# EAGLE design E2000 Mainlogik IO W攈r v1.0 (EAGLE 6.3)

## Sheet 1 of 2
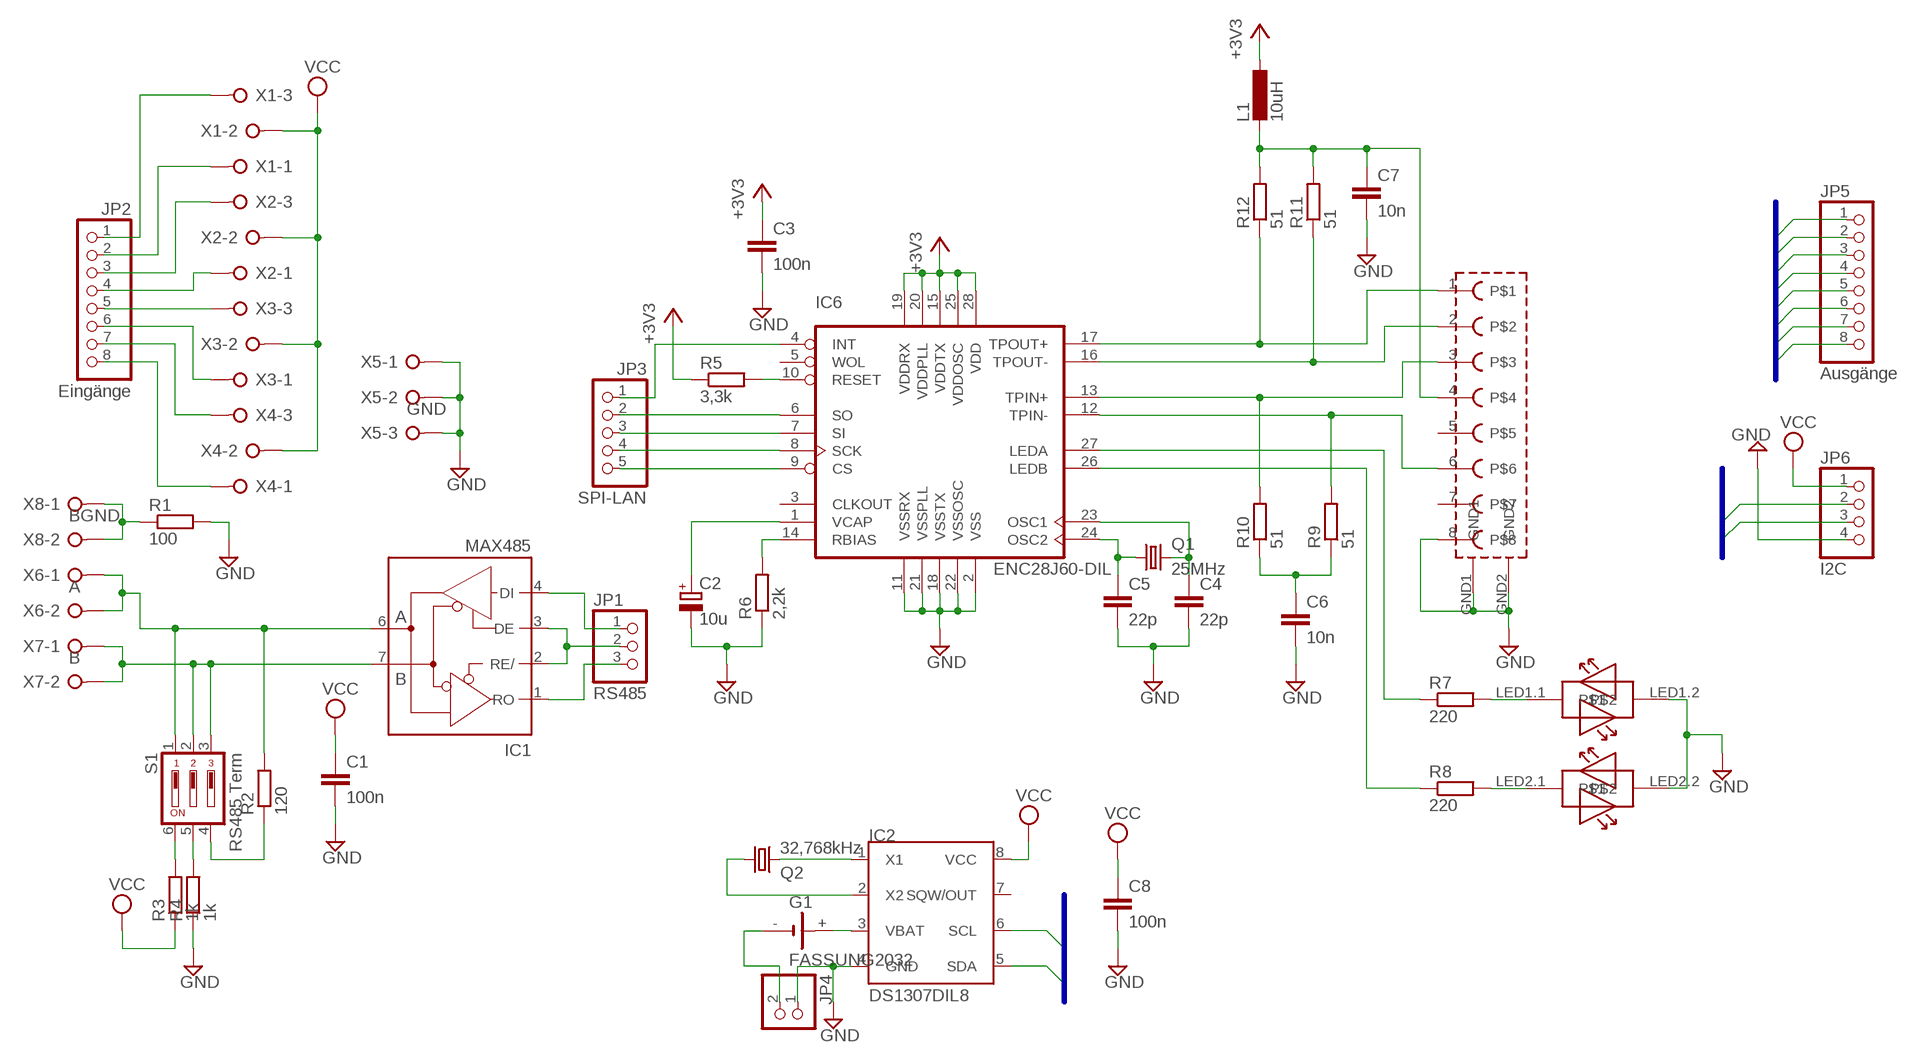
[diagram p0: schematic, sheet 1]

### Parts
C1  100n  C-EU050-025X075  [C050-025X075]
C2  10u  CPOL-EUE5-6  [E5-6]
C3  100n  C-EUC1206  [C1206]
C4  22p  C-EUC1206  [C1206]
C5  22p  C-EUC1206  [C1206]
C6  10n  C-EUC1206  [C1206]
C7  10n  C-EUC1206  [C1206]
C8  100n  C-EU050-025X075  [C050-025X075]
G1  FASSUNG2032  [BATTERY_1236_C]
IC1  MAX485  MAX481CPA  [DIL08]
IC2  DS1307DIL8  [DIL08]
IC6  ENC28J60-DIL  [DIL28-3]
J4  MAGJACK  [MAGJACK]
JP1  RS485  PINHD-1X3  [1X03]
JP2  Eingänge  PINHD-1X8  [1X08]
JP3  SPI-LAN  PINHD-1X5  [1X05]
JP4  PINHD-1X2  [1X02]
JP5  Ausgänge  PINHD-1X8  [1X08]
JP6  I2C  PINHD-1X4  [1X04]
L1  10uH  L-EUL1206  [C1206]
Q1  25MHz  CRYSTALHC49S  [HC49/S]
Q2  32,768kHz  CRYSTALTC38H  [TC38H]
R1  100  R-EU_0207/10  [0207/10]
R2  120  R-EU_0207/10  [0207/10]
R3  1k  R-EU_0207/10  [0207/10]
R4  1k  R-EU_0207/10  [0207/10]
R5  3,3k  R-EU_R1206  [R1206]
R6  2,2k  R-EU_R1206  [R1206]
R7  220  R-EU_R1206  [R1206]
R8  220  R-EU_R1206  [R1206]
R9  51  R-EU_R1206  [R1206]
R10  51  R-EU_R1206  [R1206]
R11  51  R-EU_R1206  [R1206]
R12  51  R-EU_R1206  [R1206]
S1  RS485 Term  DIP03YL  [DIP03YL]
X1  W237-3E  [W237-3E]
X2  W237-3E  [W237-3E]
X3  W237-3E  [W237-3E]
X4  W237-3E  [W237-3E]
X5  GND  W237-3E  [W237-3E]
X6  A  W237-02P  [W237-132]
X7  B  W237-02P  [W237-132]
X8  BGND  W237-02P  [W237-132]

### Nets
+3V3: C3.1 IC6.15(VDDTX) IC6.19(VDDRX) IC6.20(VDDPLL) IC6.25(VDDOSC) IC6.28(VDD) L1.1 R5.1 ; also sheet 2
A1: JP5.1 ; also sheet 2
A2: JP5.2 ; also sheet 2
A3: JP5.3 ; also sheet 2
A4: JP5.4 ; also sheet 2
A5: JP5.5 ; also sheet 2
A6: JP5.6 ; also sheet 2
A7: JP5.7 ; also sheet 2
A8: JP5.8 ; also sheet 2
CS: IC6.9(CS) JP3.5
GND: C1.2 C2.- C3.2 C4.2 C5.2 C6.2 C7.2 C8.2 IC2.4(GND) IC6.2(VSS) IC6.11(VSSRX) IC6.18(VSSTX) IC6.21(VSSPLL) IC6.22(VSSOSC) J4.8 J4.GND1 J4.GND2 J4.LED1.2 J4.LED2.2 JP4.1 JP6.4 R1.2 R4.1 R6.1 X5.1 X5.2 X5.3 ; also sheet 2
INT: IC6.4(INT) JP3.1
MISO: IC6.6(SO) JP3.2
MOSI: IC6.7(SI) JP3.3
N$1: R1.1 X8.1 X8.2
N$2: IC1.6(A) R2.2 S1.1 X6.1 X6.2
N$3: IC1.7(B) S1.2 S1.3 X7.1 X7.2
N$4: R2.1 S1.4
N$5: IC2.1(X1) Q2.2
N$6: R4.2 S1.5
N$7: R3.2 S1.6
N$8: IC2.2(X2) Q2.1
N$9: G1.+ IC2.3(VBAT)
N$10: JP2.5 X3.3
N$11: JP2.4 X2.1
N$12: JP2.3 X2.3
N$13: JP2.2 X1.1
N$14: JP2.1 X1.3
N$15: JP2.6 X3.1
N$16: JP2.7 X4.3
N$17: JP2.8 X4.1
N$18: G1.- JP4.2
N$19: IC6.10(RESET) R5.2
N$25: IC6.14(RBIAS) R6.2
N$26: C2.+ IC6.1(VCAP)
N$28: C5.1 IC6.24(OSC2) Q1.1
N$29: C4.1 IC6.23(OSC1) Q1.2
N$32: C7.1 J4.4 L1.2 R11.2 R12.2
N$33: IC6.13(TPIN+) J4.3 R10.2
N$34: J4.LED1.1 R7.2
N$35: J4.LED2.1 R8.2
N$36: IC6.12(TPIN-) J4.6 R9.2
N$37: IC6.27(LEDA) R7.1
N$38: IC6.26(LEDB) R8.1
N$41: IC6.16(TPOUT-) J4.2 R11.1
N$42: IC6.17(TPOUT+) J4.1 R12.1
N$43: C6.1 R9.1 R10.1
RX: IC1.1(RO) JP1.3
SCK: IC6.8(SCK) JP3.4
SCL: IC2.6(SCL) JP6.2 ; also sheet 2
SDA: IC2.5(SDA) JP6.3 ; also sheet 2
SEL: IC1.2(RE/) IC1.3(DE) JP1.2
TX: IC1.4(DI) JP1.1
VCC: C1.1 C8.1 IC2.8(VCC) JP6.1 R3.1 X1.2 X2.2 X3.2 X4.2 ; also sheet 2
Unconnected: IC2.7(SQW/OUT) IC6.3(CLKOUT) IC6.5(WOL) J4.5 J4.7

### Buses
SCL,SDA
A1,A2,A3,A4,A5,A6,A7,A8

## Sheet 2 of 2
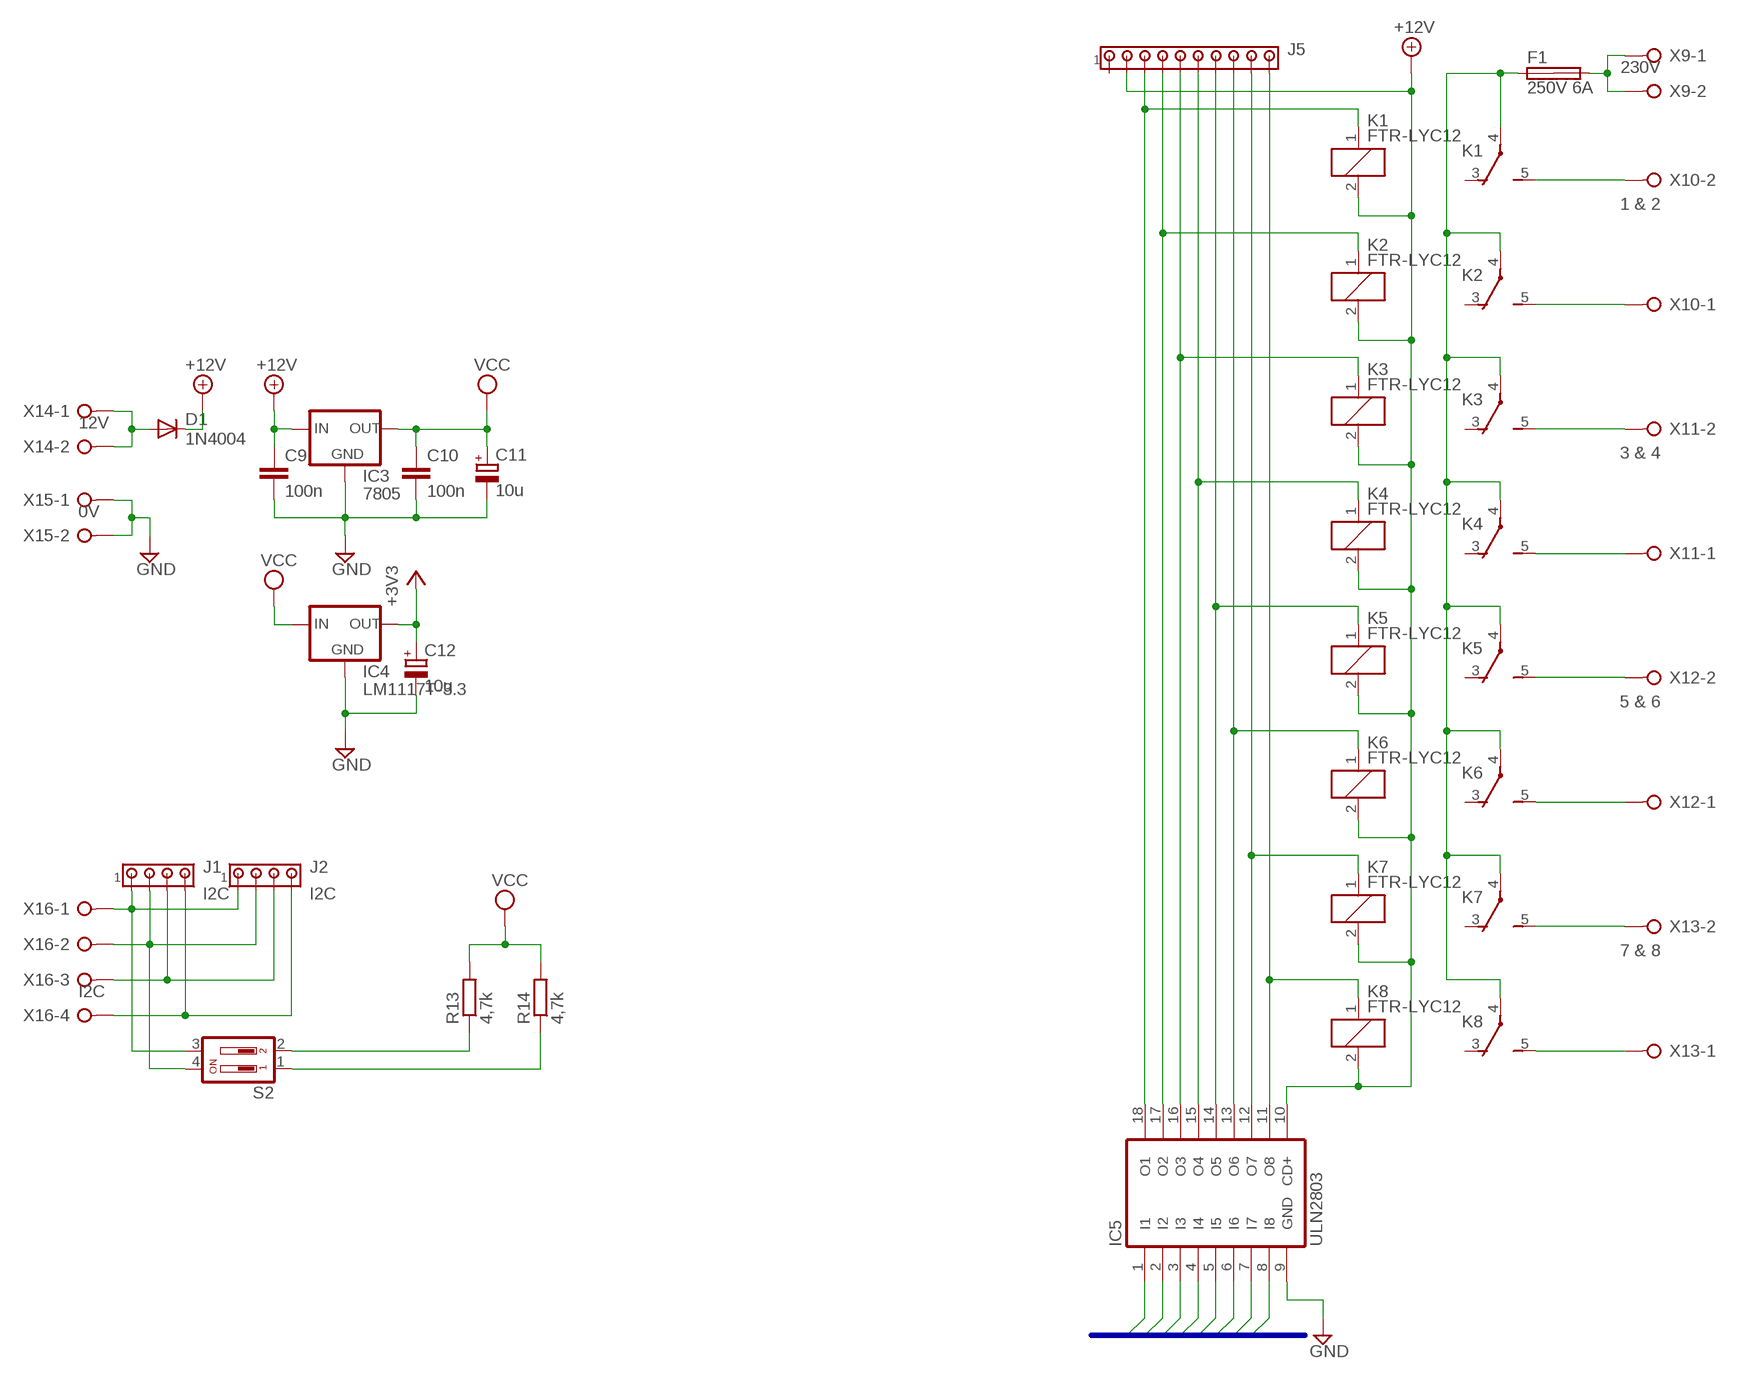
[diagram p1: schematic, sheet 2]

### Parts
C9  100n  C-EU050-025X075  [C050-025X075]
C10  100n  C-EU050-025X075  [C050-025X075]
C11  10u  CPOL-EUE5-6  [E5-6]
C12  10u  CPOL-EUE5-6  [E5-6]
D1  1N4004  [DO41-10]
F1  250V 6A  SHK20L  [SHK20L]
IC3  7805  78XXL  [78XXL]
IC4  LM1117T-3.3  [TO220]
IC5  ULN2803  ULN2803A  [DIL18]
J1  I2C  MTA04-100  [10X04MTA]
J2  I2C  MTA04-100  [10X04MTA]
J5  MTA10-100  [10X10MTA]
K1  FTR-LYC12  [FTR-LYC]
K2  FTR-LYC12  [FTR-LYC]
K3  FTR-LYC12  [FTR-LYC]
K4  FTR-LYC12  [FTR-LYC]
K5  FTR-LYC12  [FTR-LYC]
K6  FTR-LYC12  [FTR-LYC]
K7  FTR-LYC12  [FTR-LYC]
K8  FTR-LYC12  [FTR-LYC]
R13  4,7k  R-EU_0207/10  [0207/10]
R14  4,7k  R-EU_0207/10  [0207/10]
S2  DIP02YL  [DIP02YL]
X9  230V  W237-02P  [W237-132]
X10  1 & 2  W237-02P  [W237-132]
X11  3 & 4  W237-02P  [W237-132]
X12  5 & 6  W237-02P  [W237-132]
X13  7 & 8  W237-02P  [W237-132]
X14  12V  W237-02P  [W237-132]
X15  0V  W237-02P  [W237-132]
X16  I2C  W237-04P  [W237-4P]

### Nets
+3V3: C12.+ IC4.2(OUT) ; also sheet 1
+12V: C9.1 D1.C IC3.IN IC5.10(CD+) J5.2 K1.2 K2.2 K3.2 K4.2 K5.2 K6.2 K7.2 K8.2
A1: IC5.1(I1) ; also sheet 1
A2: IC5.2(I2) ; also sheet 1
A3: IC5.3(I3) ; also sheet 1
A4: IC5.4(I4) ; also sheet 1
A5: IC5.5(I5) ; also sheet 1
A6: IC5.6(I6) ; also sheet 1
A7: IC5.7(I7) ; also sheet 1
A8: IC5.8(I8) ; also sheet 1
GND: C9.2 C10.2 C11.- C12.- IC3.GND IC4.1(GND) IC5.9(GND) J1.4 J2.4 X15.1 X15.2 X16.4 ; also sheet 1
N$20: F1.2A X9.1 X9.2
N$21: F1.1A K1.4(-1:P) K2.4(-1:P) K3.4(-1:P) K4.4(-1:P) K5.4(-1:P) K6.4(-1:P) K7.4(-1:P) K8.4(-1:P)
N$22: K1.5(-1:S) X10.2
N$23: K2.5(-1:S) X10.1
N$24: K8.5(-1:S) X13.1
N$27: K7.5(-1:S) X13.2
N$30: K6.5(-1:S) X12.1
N$31: K5.5(-1:S) X12.2
N$39: K4.5(-1:S) X11.1
N$40: K3.5(-1:S) X11.2
N$44: D1.A X14.1 X14.2
N$45: IC5.11(O8) J5.10 K8.1
N$46: IC5.12(O7) J5.9 K7.1
N$47: IC5.13(O6) J5.8 K6.1
N$48: IC5.14(O5) J5.7 K5.1
N$49: IC5.15(O4) J5.6 K4.1
N$50: IC5.16(O3) J5.5 K3.1
N$51: IC5.17(O2) J5.4 K2.1
N$52: IC5.18(O1) J5.3 K1.1
N$53: R13.1 S2.2
N$54: R14.1 S2.1
SCL: J1.1 J2.1 S2.3 X16.1 ; also sheet 1
SDA: J1.2 J2.2 S2.4 X16.2 ; also sheet 1
VCC: C10.1 C11.+ IC3.OUT IC4.3(IN) J1.3 J2.3 R13.2 R14.2 X16.3 ; also sheet 1
Unconnected: F1.1B F1.2B J5.1 K1.3(-1:O) K2.3(-1:O) K3.3(-1:O) K4.3(-1:O) K5.3(-1:O) K6.3(-1:O) K7.3(-1:O) K8.3(-1:O)

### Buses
A1,A2,A3,A4,A5,A6,A7,A8

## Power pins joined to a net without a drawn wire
GND: IC1.5(GND)
VCC: IC1.8(VCC)

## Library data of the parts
C1 C3-C10 = rcl:C-EU: CAPACITOR, European symbol
C2 C11 C12 = rcl:CPOL-EU: POLARIZED CAPACITOR, European symbol
D1 = diode:1N4004: DIODE
F1 = fuse:SHK20L: FUSE HOLDER 5 x 20 mm, SH contact, SHH1 Schukat, E1073 Buerklin; OC_FARNELL: unknown; OC_NEWARK: unknown
G1 = battery:FASSUNG2032: LI BATTERY Sonnenschein
IC1 = maxim:MAX481CPA: RS485 TRANSEIVER; MPN: MAX481CPA+; OC_FARNELL: unknown; OC_NEWARK: 99K3445
IC2 = dallas:DS1307: I2C Serial RTC w/56 bytes battery backed RAM
IC3 = v-reg:78XXL: VOLTAGE REGULATOR
IC4 = lm1117:LM1117T-*
IC5 = uln-udn:ULN2803A: DRIVER ARRAY
IC6 = enc28j60centered:ENC28J60-*: Microchip 10Mbit Ethernet controller with SPI interface Improved SOIC28 layout (pads in 0.01 raster, pin1 slightly smaller). Pin 6 (SO) changed from Out (paralleling several Outs gives an error) to OC. Author: Profi from mikrocontroller.net - forum Date: 2006.0827
J1 J2 = con-amp:MTA04-100: AMP connector
J4 = magjacksmalldrill:MAGJACK
J5 = con-amp:MTA10-100: AMP connector
JP1 = pinhead:PINHD-1X3: PIN HEADER
JP2 JP5 = pinhead:PINHD-1X8: PIN HEADER
JP3 = pinhead:PINHD-1X5: PIN HEADER
JP4 = pinhead:PINHD-1X2: PIN HEADER
JP6 = pinhead:PINHD-1X4: PIN HEADER
K1-K8 = relay:FTR-LYC: Schmales Netzrelais NETZRELAIS FTR-LYCA024V 1XUM 6A/250VAC Distributor: Conrad electronic Bestell Nr.: 504382 - 62 Source: http://www2.produktinfo.conrad.com/datenblaetter/500000-524999/504382-da-01-de-NETZRELAIS_FTR-LYCA024V_1XUM_6A_250VAC.pdf; OC_FARNELL: unknown; OC_NEWARK: unknown
L1 = rcl:L-EU: INDUCTOR, European symbol
Q1 = crystal:CRYSTAL: CRYSTAL; OC_FARNELL: 1667008; OC_NEWARK: unknown
Q2 = crystal:CRYSTAL: CRYSTAL; OC_FARNELL: unknown; OC_NEWARK: unknown
R1-R14 = rcl:R-EU_: RESISTOR, European symbol
S1 = switch-dil:DIP03YL: DIL/CODE SWITCH; OC_FARNELL: unknown; OC_NEWARK: unknown
S2 = switch-dil:DIP02YL: DIL/CODE SWITCH; OC_FARNELL: unknown; OC_NEWARK: unknown
X1-X5 = con-wago-508:W237-3E: WAGO SREW CLAMP; OC_FARNELL: unknown; OC_NEWARK: unknown
X6-X15 = con-wago-508:W237-02P: WAGO SREW CLAMP; OC_FARNELL: unknown; OC_NEWARK: unknown
X16 = con-wago-508:W237-04P: WAGO SREW CLAMP; OC_FARNELL: unknown; OC_NEWARK: unknown

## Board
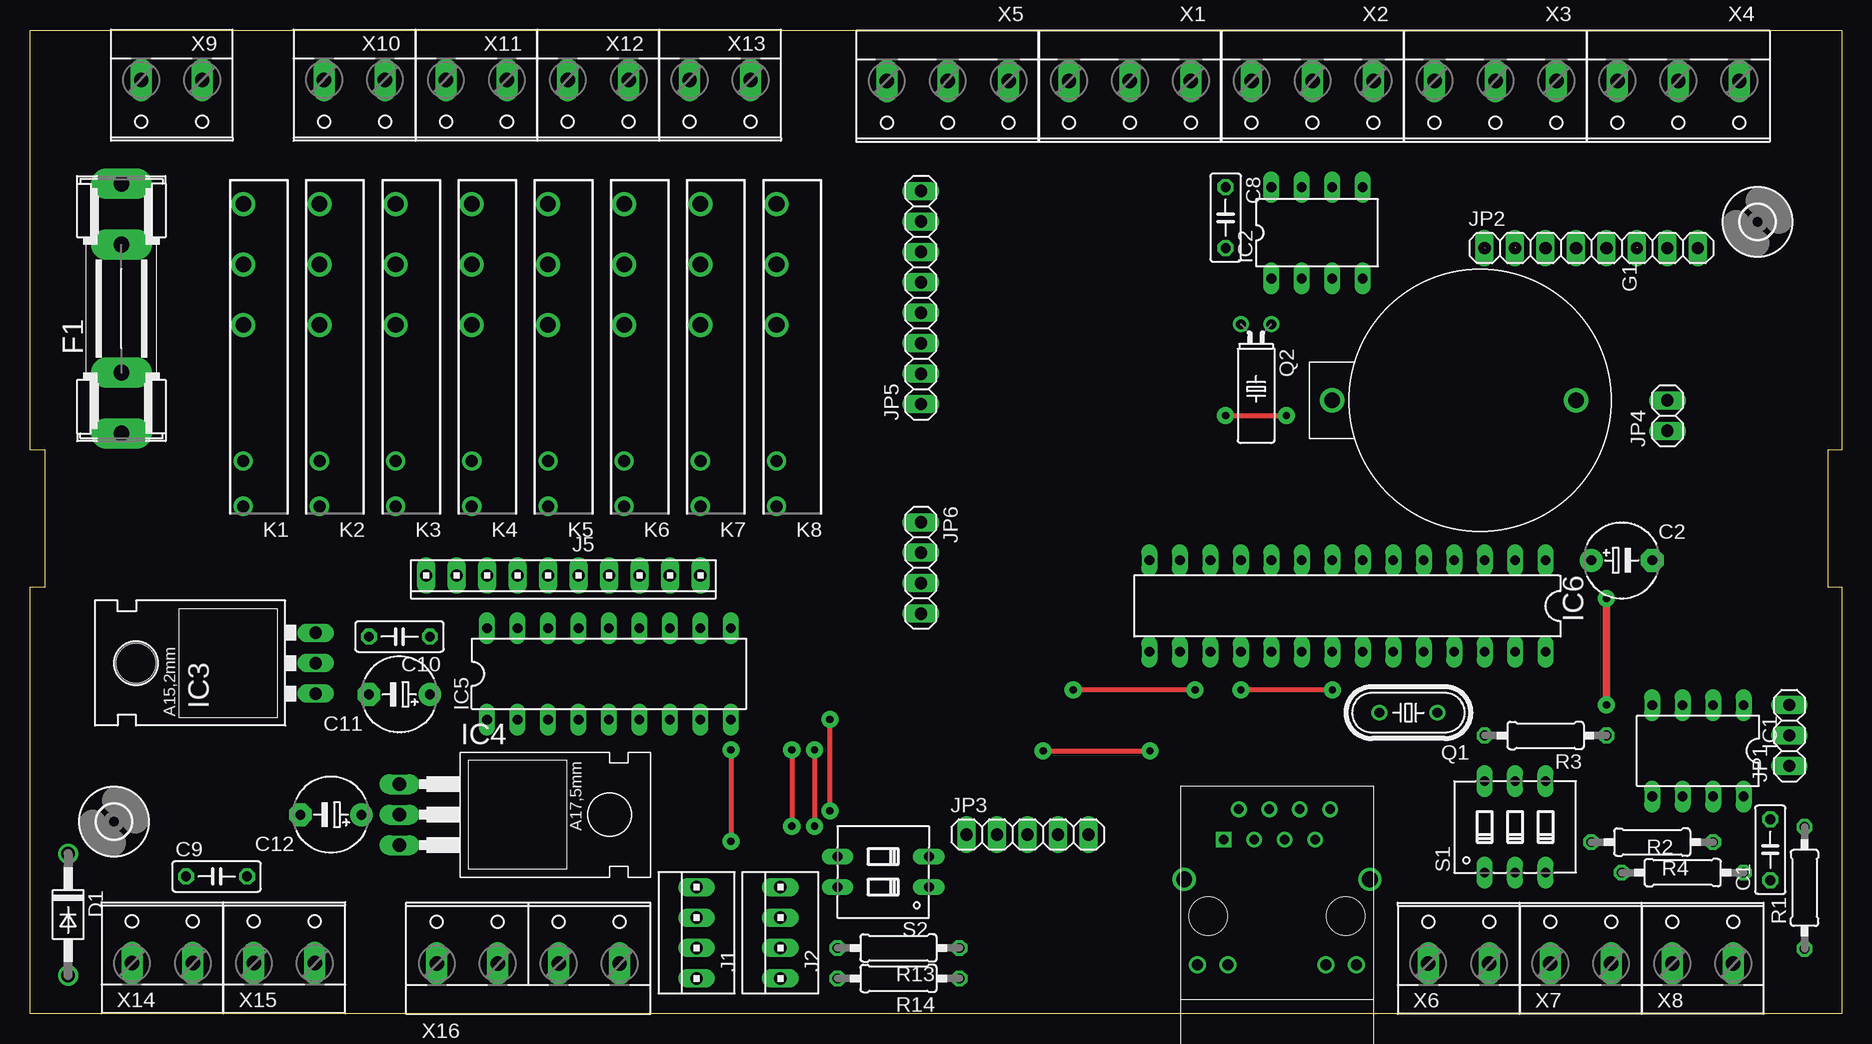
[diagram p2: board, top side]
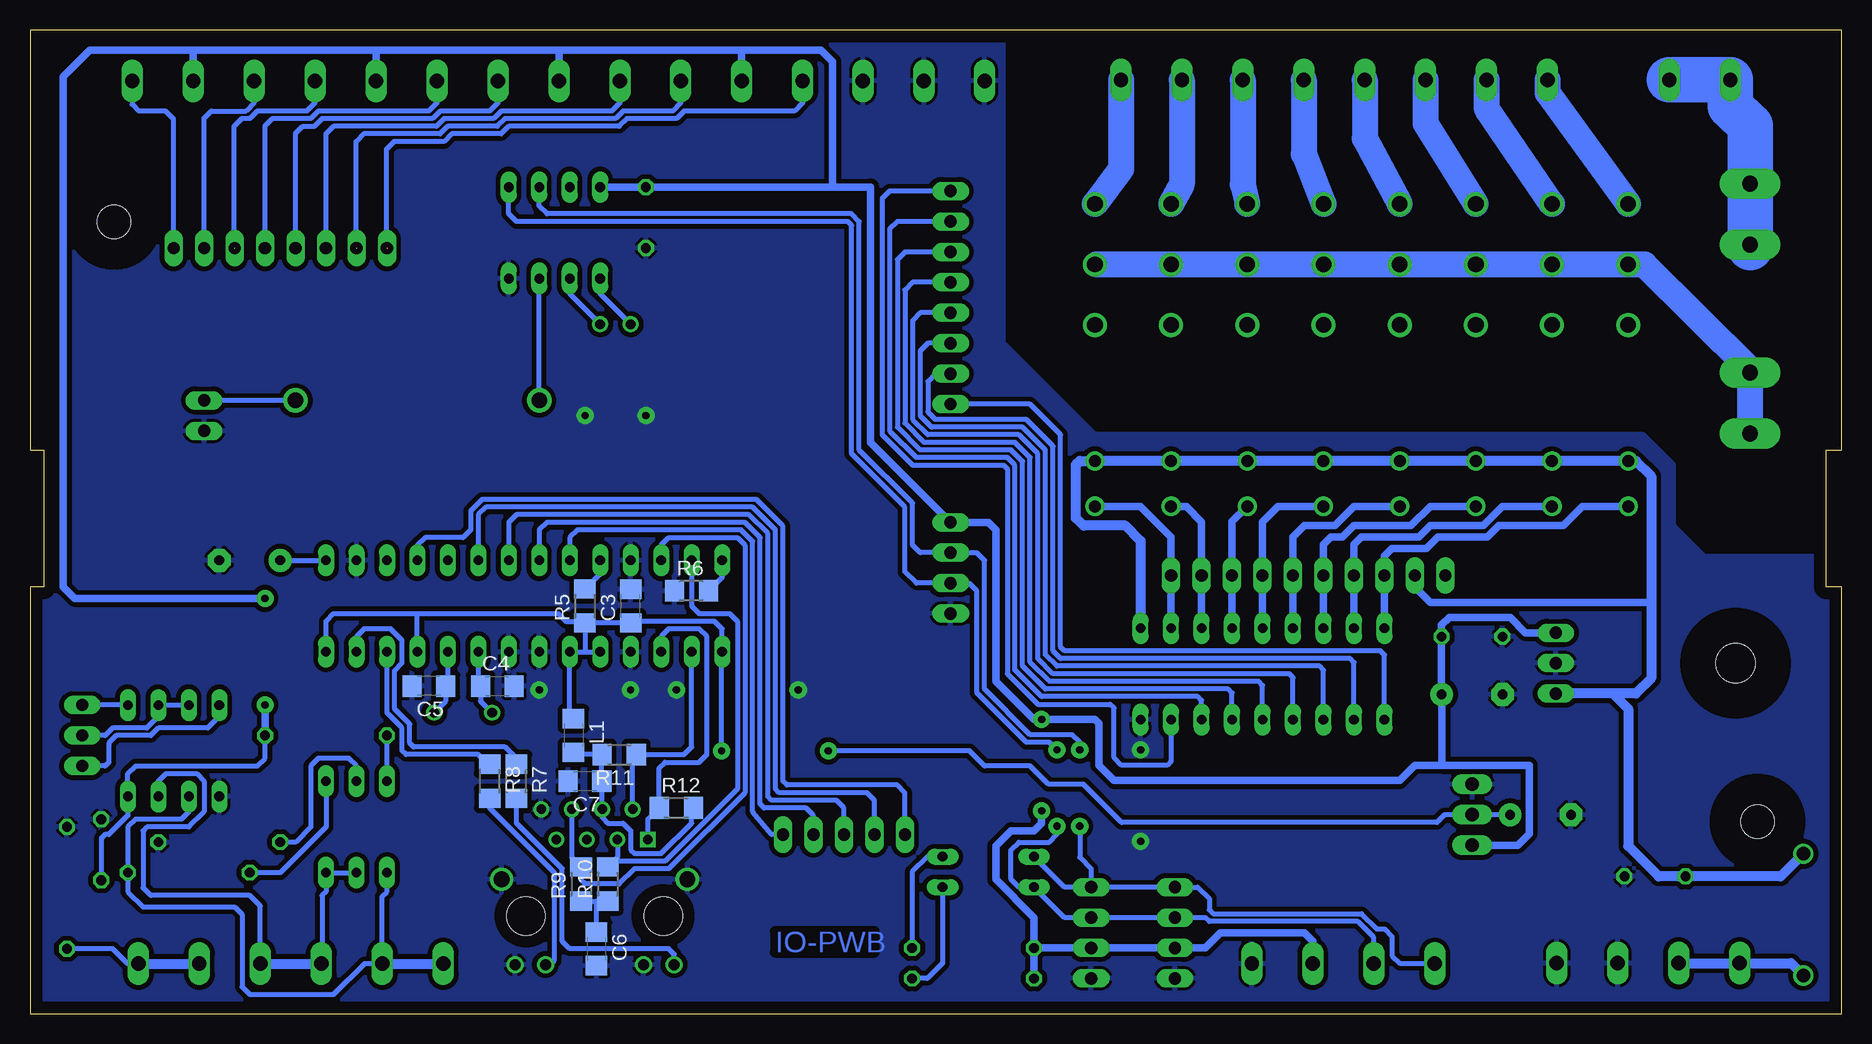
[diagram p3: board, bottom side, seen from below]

Size 151 x 82 mm. Coordinates in mm from the lower left corner, seen from the top.
Outline: 0,0 0,35.56 1.27,35.56 1.27,46.99 0,46.99 0,82 151,82 151,46.99 149.86,46.99 149.86,35.56 151,35.56 151,0 0,0
Copper layers (1*16): Top 0.035mm / dielectric 1.5mm / Bottom 0.035mm
Design rules "default": minimum track width 10mil, minimum drill 24mil, track to track 8mil, track to pad 8mil, pad to pad 8mil, via to via 8mil, smd to smd 8mil, copper to edge 40mil, drill to drill 8mil, minimum pad ring 10mil, minimum via ring 8mil, stop-mask expansion 4mil, vias tented up to drill 0mil, thermal gap 10mil

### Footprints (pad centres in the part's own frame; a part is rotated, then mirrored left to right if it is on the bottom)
C050-025X075 = drill 0.813 octagon: 1 -2.54,0; 2 2.54,0
E5-6 = drill 0.813 pad 1.905: + -2.54,0 | drill 0.813 pad 1.905 octagon: - 2.54,0
C1206 = smd 1.6 x 1.8: 1 -1.4,0; 2 1.4,0
DO41-10 = drill 1.118: A 5.08,0; C -5.08,0
SHK20L = drill 1.321 pad 2.54 long: 1A -10.414,0; 1B -5.334,0; 2A 10.414,0; 2B 5.334,0
BATTERY_1236_C = drill 1.27 pad 2.032: + 0,0; - 0,20.32
DIL08 = drill 0.813 long: 1 -3.81,-3.81; 2 -1.27,-3.81; 3 1.27,-3.81; 4 3.81,-3.81; 5 3.81,3.81; 6 1.27,3.81; 7 -1.27,3.81; 8 -3.81,3.81
78XXL = drill 1.016 long: GND 0,-3.81; IN -2.54,-3.81; OUT 2.54,-3.81 | hole 3.302: 0,11.176
TO220 = drill 1.118 long: 1 -2.54,-6.35; 2 0,-6.35; 3 2.54,-6.35
DIL18 = drill 0.813 long: 1 -10.16,-3.81; 2 -7.62,-3.81; 3 -5.08,-3.81; 4 -2.54,-3.81; 5 0,-3.81; 6 2.54,-3.81; 7 5.08,-3.81; 8 7.62,-3.81; 9 10.16,-3.81; 10 10.16,3.81; 11 7.62,3.81; 12 5.08,3.81; 13 2.54,3.81; 14 0,3.81; 15 -2.54,3.81; 16 -5.08,3.81; 17 -7.62,3.81; 18 -10.16,3.81
DIL28-3 = drill 0.813 long: 1 -16.51,-3.81; 2 -13.97,-3.81; 3 -11.43,-3.81; 4 -8.89,-3.81; 5 -6.35,-3.81; 6 -3.81,-3.81; 7 -1.27,-3.81; 8 1.27,-3.81; 9 3.81,-3.81; 10 6.35,-3.81; 11 8.89,-3.81; 12 11.43,-3.81; 13 13.97,-3.81; 14 16.51,-3.81; 15 16.51,3.81; 16 13.97,3.81; 17 11.43,3.81; 18 8.89,3.81; 19 6.35,3.81; 20 3.81,3.81; 21 1.27,3.81; 22 -1.27,3.81; 23 -3.81,3.81; 24 -6.35,3.81; 25 -8.89,3.81; 26 -11.43,3.81; 27 -13.97,3.81; 28 -16.51,3.81
10X04MTA = drill 1.016 long: 1 3.81,0; 2 1.27,0; 3 -1.27,0; 4 -3.81,0
MAGJACK = drill 0.8 square: 1 -4.445,6.35 | drill 0.8: 2 -3.175,8.89; 3 -1.905,6.35; 4 -0.635,8.89; 5 0.635,6.35; 6 1.905,8.89; 7 3.175,6.35; 8 4.445,8.89 | drill 1.3: GND1 -7.747,3.048; GND2 7.747,3.048 | drill 0.9: LED1.1 -6.629,-4.064; LED1.2 -4.089,-4.064; LED2.1 4.089,-4.064; LED2.2 6.629,-4.064 | hole 3.2: -5.715,0; 5.715,0
10X10MTA = drill 1.016 long: 1 11.43,0; 2 8.89,0; 3 6.35,0; 4 3.81,0; 5 1.27,0; 6 -1.27,0; 7 -3.81,0; 8 -6.35,0; 9 -8.89,0; 10 -11.43,0
1X03 = drill 1.016 long: 1 -2.54,0; 2 0,0; 3 2.54,0
1X08 = drill 1.016 long: 1 -8.89,0; 2 -6.35,0; 3 -3.81,0; 4 -1.27,0; 5 1.27,0; 6 3.81,0; 7 6.35,0; 8 8.89,0
1X05 = drill 1.016 long: 1 -5.08,0; 2 -2.54,0; 3 0,0; 4 2.54,0; 5 5.08,0
1X02 = drill 1.016 long: 1 -1.27,0; 2 1.27,0
1X04 = drill 1.016 long: 1 -3.81,0; 2 -1.27,0; 3 1.27,0; 4 3.81,0
FTR-LYC = drill 1 pad 1.6: 1 -3.78,0; 2 0,0 | drill 1.3 pad 2: 3 11.34,0; 4 16.38,0; 5 21.42,0
HC49/S = drill 0.813: 1 -2.413,0; 2 2.413,0
TC38H = drill 0.813: 1 -1.27,0; 2 1.27,0
0207/10 = drill 0.813 octagon: 1 -5.08,0; 2 5.08,0
R1206 = smd 1.6 x 1.803: 1 -1.422,0; 2 1.422,0
DIP03YL = drill 0.813 long: 1 -2.54,-3.81; 2 0,-3.81; 3 2.54,-3.81; 4 2.54,3.81; 5 0,3.81; 6 -2.54,3.81
DIP02YL = drill 0.813 long: 1 -1.27,-3.81; 2 1.27,-3.81; 3 1.27,3.81; 4 -1.27,3.81
2,8 = hole 2.8: 0,0
W237-3E = drill 1.194 long: 1 -5.08,-0.635; 2 0,-0.635; 3 5.08,-0.635
W237-132 = drill 1.194 long: 1 -2.54,-0.635; 2 2.54,-0.635
W237-4P = drill 1.194 long: 1 -7.62,-0.635; 2 -2.54,-0.635; 3 2.54,-0.635; 4 7.62,-0.635

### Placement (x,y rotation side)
C1  145.06,13.65 90 top
C2  132.68,37.78 0 top
C3  100.93,33.97 90 bottom
C4  112.04,27.3 0 bottom
C5  117.76,27.3 180 bottom
C6  103.79,5.4 270 bottom
C7  104.74,19.37 180 bottom
C8  99.66,66.36 270 top
C9  15.55,11.43 0 top
C10  30.8,31.43 180 top
C11  30.79,26.6 180 top
C12  25.08,16.57 180 top
D1  3.17,8.25 270 top
F1  7.62,58.77 90 top
G1  108.55,51.12 270 top
IC1  139.03,21.91 180 top
IC2  107.28,65.09 0 top
IC3  20.01,29.21 90 top
IC4  37.14,16.58 270 top
IC5  48.26,28.32 0 top
IC6  109.82,33.97 180 top
J1  55.56,6.73 90 top
J2  62.55,6.73 90 top
J4  103.94,8.14 0 top
J5  44.45,36.51 180 top
JP1  146.65,23.18 90 top
JP2  130.14,63.82 0 top
JP3  83.15,14.92 0 top
JP4  136.49,49.85 90 top
JP5  74.26,59.69 90 top
JP6  74.26,37.15 270 top
K1  17.78,46.07 90 top
K2  24.13,46.07 90 top
K3  30.48,46.07 90 top
K4  36.83,46.07 90 top
K5  43.18,46.07 90 top
K6  49.53,46.07 90 top
K7  55.88,46.07 90 top
K8  62.23,46.07 90 top
L1  105.69,23.18 270 bottom
Q1  114.9,25.08 180 top
Q2  102.2,57.47 180 top
R1  147.92,10.48 90 top
R2  137.76,11.75 0 top
R3  126.33,23.18 180 top
R4  135.22,14.29 180 top
R5  104.74,33.97 90 bottom
R6  95.85,35.24 0 bottom
R7  110.45,19.37 270 bottom
R8  112.68,19.37 270 bottom
R9  105.06,10.79 90 bottom
R10  102.83,10.79 90 bottom
R11  101.88,21.59 180 bottom
R12  97.12,17.14 0 bottom
R13  72.39,5.46 180 top
R14  72.39,2.92 180 top
S1  123.79,15.56 0 top
S2  71.12,11.81 90 top
U$2  [2,8]  7,16 0 top
U$3  [2,8]  144,66 0 top
X1  91.68,77.13 180 top
X2  106.91,77.13 180 top
X3  122.16,77.13 180 top
X4  137.4,77.13 180 top
X5  76.5,77.12 180 top
X6  119.09,4.8 0 top
X7  129.26,4.8 0 top
X8  139.43,4.8 0 top
X9  11.81,77.2 180 top
X10  27.05,77.21 180 top
X11  37.21,77.2 180 top
X12  47.37,77.2 180 top
X13  57.52,77.2 180 top
X14  11.04,4.83 0 top
X15  21.2,4.83 0 top
X16  41.53,4.8 0 top

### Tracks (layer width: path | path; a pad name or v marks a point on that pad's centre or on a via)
+3V3  (via drill 0.6 pad 1.42)
  Top 0.406: v84.45,21.91 v93.34,21.91
  Bottom 0.406: 104.74,30.16 IC6.20 106.01,24.45 105.88,24.58 L1.1 | 104.74,30.16 IC6.19 | R5.1 104.74,30.16 | R5.1 104.72,32.57 C3.1 100.8,32.7 93.94,32.7 93.31,32.07 IC6.15 93.34,30.13 v93.34,21.91 | IC6.28 126.33,32.7 125.69,33.34 118.71,33.34 | 118.71,33.34 106.96,33.34 106.33,32.7 104.89,32.7 R5.1 | IC6.25 118.71,33.34 | C12.+ IC4.2 33.09,16.58 33.72,15.94 60.01,15.94 63.18,19.11 66.1,19.11 67.63,20.64 71.44,20.64 72.71,21.91 v84.45,21.91
+12V
  Bottom 0.61: J5.2 35.56,35.56 34.29,34.29 15.88,34.29
  Bottom 0.813: D1.C 3.18,13.33 5.08,11.43 C9.1 15.24,11.43 17.78,13.97 17.78,25.4 19.05,26.67 | 19.05,26.67 17.14,26.67 15.88,27.94 15.88,34.29 15.88,44.8 17.14,46.07 K1.2 K2.2 K3.2 K4.2 K5.2 K6.2 K7.2 K8.2 63.5,46.07 63.82,45.75 63.82,41.31 63.18,40.67 59.69,40.67 58.42,39.4 IC5.10 | 19.05,26.67 IC3.IN
A1
  Bottom 0.406: IC5.1 38.1,29.91 38.42,30.23 64.77,30.23 65.09,30.55 65.09,48.26 67.63,50.8 JP5.1
A2
  Bottom 0.406: JP5.2 75.53,53.34 76.17,52.7 76.17,50.16 75.53,49.53 67.94,49.53 65.72,47.31 65.72,30.23 65.09,29.6 40.96,29.6 40.64,29.28 IC5.2
A3
  Bottom 0.406: JP5.3 76.17,55.88 76.8,55.24 76.8,49.85 75.85,48.9 68.26,48.9 66.36,46.99 66.36,29.91 65.41,28.96 43.5,28.96 43.18,28.64 IC5.3
A4
  Bottom 0.406: JP5.4 76.8,58.42 77.44,57.78 77.44,49.53 76.17,48.26 68.58,48.26 66.99,46.67 66.99,29.6 65.72,28.33 46.04,28.33 45.72,28.01 IC5.4
A5
  Bottom 0.406: JP5.5 77.44,60.96 78.07,60.33 78.07,49.21 76.48,47.62 68.9,47.62 67.63,46.35 67.63,29.28 66.04,27.69 48.58,27.69 48.26,27.38 IC5.5
A6
  Bottom 0.406: JP5.6 78.07,63.5 78.7,62.87 78.7,48.9 76.8,46.99 69.22,46.99 68.26,46.04 68.26,28.96 66.36,27.06 51.12,27.06 50.8,26.74 IC5.6
A7
  Bottom 0.406: JP5.7 78.7,66.04 79.34,65.41 79.34,48.58 77.12,46.35 69.53,46.35 68.9,45.72 68.9,28.64 66.67,26.42 53.66,26.42 53.34,26.11 IC5.7
A8
  Bottom 0.406: JP5.8 79.34,68.58 79.97,67.94 79.97,48.26 77.44,45.72 69.85,45.72 69.53,45.4 69.53,28.33 66.99,25.79 60.96,25.79 60.64,25.47 60.64,21.34 60.01,20.71 56.2,20.71 55.88,21.02 IC5.8
CS
  Bottom 0.406: JP3.5 89.18,14.92 90.77,16.83 90.77,39.37 91.72,40.32 105.38,40.32 106.01,39.69 IC6.9
GND  (via drill 0.6 pad 1.42)
  Top 0.406: v108.55,26.99 v100.93,26.99 | v97.12,26.99 v86.96,26.99 | v99.66,49.85 v104.74,49.85 | v58.42,21.97 v58.42,14.35
  pour Bottom (isolate 0.406): -1.27,38.1 11.43,38.1 13.97,40.64 13.97,45.72 16.51,48.26 62.23,48.26 69.85,55.88 69.85,82.55 152.4,82.55 152.4,-1.27 -1.27,-1.27
INT
  Bottom 0.406: IC6.4 118.71,39.05 118.08,39.69 114.9,39.69 114.27,40.32 114.27,41.91 113.31,42.86 90.45,42.86 88.23,40.64 88.23,19.37 87.91,19.05 78.7,19.05 78.07,18.41 JP3.1
MISO
  Bottom 0.406: JP3.2 80.61,17.78 81.25,18.41 88.55,18.41 88.86,18.73 88.86,40.32 90.77,42.23 113,42.23 113.63,41.59 IC6.6
MOSI
  Bottom 0.406: JP3.3 83.15,17.14 83.78,17.78 89.18,17.78 89.5,18.1 89.5,40.01 91.09,41.59 110.45,41.59 111.09,40.96 IC6.7
N$1
  Bottom 0.406: X8.2 142.88,4.16 144.11,5.4 R1.1
  Bottom 0.813: X8.2 X8.1
N$2
  Bottom 0.406: IC1.6 137.76,16.83 138.4,16.19 142.21,16.19 142.84,15.56 R2.2 142.84,10.16 141.57,8.89 133.95,8.89 133.31,8.26 133.31,2.22 132.68,1.59 125.69,1.59 123.12,4.16 X6.2 121.63,9.78 121.25,10.16 S1.1
  Bottom 0.813: X6.2 X6.1
N$3
  Bottom 0.406: IC1.7 140.3,19.37 139.66,20 137.12,20 136.49,19.37 136.49,16.83 137.76,15.56 141.25,15.56 141.57,15.24 141.57,10.48 140.94,9.84 132.68,9.84 131.8,8.96 X7.2 | S1.2 S1.3 126.33,10.16 126.65,9.84 126.65,4.24 X7.1
  Bottom 0.813: X7.2 X7.1
N$4
  Bottom 0.406: S1.4 126.33,15.56 130.14,11.75 R2.1
N$5
  Bottom 0.406: Q2.2 103.47,60.01 IC2.1
N$6
  Bottom 0.406: S1.5 123.79,20.64 124.42,21.27 126.97,21.27 127.6,20.64 127.6,15.56 128.87,14.29 R4.2
N$7
  Bottom 0.406: S1.6 R3.2
N$8
  Bottom 0.406: IC2.2 106.01,60.01 Q2.1
N$9
  Bottom 0.406: G1.+ IC2.3
N$10
  Bottom 0.406: X3.3 117.08,75.92 117.76,75.25 126.97,75.25 127.6,74.61 130.81,74.61 131.41,74.01 JP2.5
N$11
  Bottom 0.406: X2.1 111.99,75.94 112.68,75.25 116.81,75.25 117.44,74.61 126.65,74.61 127.28,73.98 128.27,73.98 128.87,73.38 JP2.4
N$12
  Bottom 0.406: X2.3 101.83,75.94 102.52,75.25 111.72,75.25 112.36,74.61 116.49,74.61 117.12,73.98 125.69,73.98 126.33,73.34 JP2.3
N$13  (1 unrouted)
  Bottom 0.406: X1.1 96.76,75.92 97.44,75.25 101.56,75.25 102.2,74.61 111.41,74.61 112.04,73.98 116.17,73.98 116.81,73.34 123.19,73.34 123.83,72.71 123.83,63.85
N$14  (1 unrouted)
  Bottom 0.406: X1.3 86.6,75.92 87.28,75.25 96.48,75.25 97.12,74.61 101.25,74.61 101.88,73.98 111.09,73.98 111.72,73.34 115.85,73.34 116.49,72.71 120.65,72.71 121.28,72.07 121.28,63.85
N$15  (1 unrouted)
  Bottom 0.406: X3.1 127.24,75.92 127.92,75.25 132.04,75.25 132.68,74.61 133.35,74.61 133.99,73.98 133.99,63.85
N$16
  Bottom 0.406: X4.3 132.32,75.92 133,75.25 135.89,75.25 136.49,74.65 JP2.7
N$17
  Bottom 0.406: JP2.8 139.03,74.58 139.7,75.25 141.92,75.25 142.48,75.81 X4.1
N$18
  Bottom 0.406: G1.- JP4.2
N$19
  Bottom 0.406: IC6.10 103.47,36.66 R5.2
N$20
  Bottom 3.81: X9.1 X9.2 9.27,75.66 7.62,74.01 F1.2A 7.62,63.85
N$21
  Bottom 0.254: K8.4 62.23,62.27 62.1,62.45
  Bottom 2.184: F1.1A 7.62,53.69 16.43,62.45 K1.4 K2.4 K3.4 K4.4 K5.4 K6.4 K7.4 62.1,62.45
N$22
  Bottom 2.184: X10.2 24.51,76.76 K1.5
N$23
  Bottom 2.184: X10.1 29.59,75.49 K2.5
N$24
  Bottom 2.184: X13.1 60.06,70.4 K8.5
N$25
  Bottom 0.406: IC6.14 93.31,36.36 R6.2
N$26
  Bottom 0.406: C2.+ IC6.1
N$27
  Bottom 2.184: X13.2 54.98,69.13 K7.5
N$28
  Bottom 0.406: IC6.24 116.17,27.49 C5.1 116.36,26.04 Q1.1
N$29
  Bottom 0.406: IC6.23 113.63,27.49 C4.1 113.44,26.04 Q1.2
N$30
  Bottom 2.184: X12.1 49.91,69.14 K6.5
N$31
  Bottom 2.184: X12.2 44.83,71.68 K5.5
N$32
  Bottom 0.406: L1.2 105.5,21.59 R11.2 103.34,21.55 C7.1 103.31,19.33 J4.4 103.31,16.34 102.83,15.88 101.56,15.88 100.93,15.24 100.93,13.65 100.61,13.34 98.39,13.34 95.85,15.88 95.85,16.99 R12.2
N$33
  Bottom 0.406: J4.3 102.03,13.02 R10.2 102.35,12.7 98.07,12.7 92.04,18.73 92.04,32.7 92.67,33.34 95.22,33.34 95.85,33.97 IC6.13
N$34
  Bottom 0.406: J4.LED1.1 97.31,4.95 97.75,5.4 106.01,5.4 106.64,6.03 106.64,12.06 110.45,15.88 R7.2
N$35
  Bottom 0.406: J4.LED2.1 107.65,4.07 107.28,4.45 107.28,11.75 112.68,17.14 R8.2
N$36
  Bottom 0.406: J4.6 105.84,13.01 R9.2 105.06,11.11 104.74,10.79 101.88,10.79 100.61,12.06 97.75,12.06 91.41,18.41 91.41,39.05 92.04,39.69 97.75,39.69 98.39,39.05 IC6.12
N$37
  Bottom 0.406: R7.1 110.45,21.27 111.41,22.23 119.03,22.23 119.34,22.54 119.34,24.13 120.61,25.4 120.61,28.57 119.98,29.21 119.98,31.11 120.93,32.07 123.16,32.07 123.79,31.43 IC6.27
N$38
  Bottom 0.406: R8.1 112.83,20.79 113.63,21.59 119.66,21.59 119.98,21.91 119.98,23.81 121.25,25.08 IC6.26
N$39
  Bottom 2.184: X11.1 39.75,72.95 K4.5
N$40
  Bottom 2.184: X11.2 34.67,74.22 K3.5
N$41
  Bottom 0.406: J4.2 100.77,21.29 R11.1 96.48,21.59 95.85,22.23 IC6.16
N$42
  Bottom 0.406: J4.1 99.5,16.19 R12.1 98.54,20.48 98.07,20.95 95.22,20.95 94.58,21.59 94.58,31.43 95.22,32.07 97.75,32.07 98.39,31.43 IC6.17
N$43
  Bottom 0.406: R9.1 103.79,9.37 | 103.79,9.37 R10.1 | C6.1 103.79,9.37
N$44
  Bottom 0.813: X14.2 X14.1 4.2,4.2 D1.A
N$45
  Bottom 0.61: K8.1 62.2,42.26 58.42,42.26 55.88,39.72 J5.10 IC5.11
N$46
  Bottom 0.61: K7.1 55.85,42.26 54.61,42.26 53.34,40.99 J5.9 IC5.12
N$47
  Bottom 0.61: K6.1 50.8,41.02 J5.8 IC5.13
N$48
  Bottom 0.61: K5.1 43.21,42.26 46.99,42.26 48.26,40.99 J5.7 IC5.14
N$49
  Bottom 0.61: K4.1 36.86,42.26 40.64,42.26 42.23,40.67 44.77,40.67 45.72,39.72 J5.6 IC5.15
N$50
  Bottom 0.61: K3.1 30.51,42.26 34.29,42.26 35.88,40.67 40.64,40.67 41.59,39.72 42.55,39.72 43.18,39.09 J5.5 IC5.16
N$51
  Bottom 0.61: K2.1 24.16,42.26 28.26,42.26 29.84,40.67 34.29,40.67 35.24,39.72 40.01,39.72 40.64,39.09 J5.4 IC5.17
N$52
  Bottom 0.61: K1.1 17.81,42.26 21.59,42.26 23.18,40.67 28.57,40.67 29.53,39.72 33.66,39.72 34.61,38.77 37.47,38.77 38.1,38.13 J5.3 IC5.18
N$53
  Bottom 0.406: S2.2 76.2,13.08 77.47,11.81 R13.1
N$54
  Bottom 0.406: S2.1 74.93,4.19 76.2,2.92 R14.1
RX
  Bottom 0.406: IC1.1 JP1.3
SCK
  Bottom 0.406: JP3.4 85.69,16.51 86.33,17.14 89.82,17.14 90.14,17.46 90.14,39.69 91.41,40.96 107.92,40.96 108.55,40.32 IC6.8
SCL  (via drill 0.6 pad 1.42)
  Top 0.406: v63.5,21.97 v63.5,15.62
  Bottom 0.406: IC2.6 108.55,67.31 107.92,66.67 82.52,66.67 81.88,66.04 81.88,46.99 77.44,42.55 77.44,39.05 76.8,38.42 JP6.2 72.07,38.42 72.07,38.41 71.44,37.77 71.44,27.05 67.63,23.24 64.14,23.24 63.5,22.61 v63.5,21.97 | J2.1 J1.1 53.66,10.54 52.7,9.59 52.7,8.63 52.39,8.32 40.01,8.32 38.73,7.05 38.1,7.05 37.47,6.41 37.47,4.83 36.83,4.19 33.94,4.19 X16.1 | J2.1 64.77,10.54 S2.3 | v63.5,15.62 63.5,13.02 62.55,12.06 J2.1
SDA  (via drill 0.6 pad 1.42)
  Top 0.406: v65.41,21.97 v65.41,15.62
  Bottom 0.406: IC2.5 111.09,66.67 110.45,66.04 82.83,66.04 82.52,65.72 82.52,46.67 78.07,42.23 78.07,36.83 77.12,35.88 JP6.3 72.71,35.88 72.71,35.87 72.07,35.23 72.07,26.73 67.94,22.61 66.04,22.61 v65.41,21.97 | X16.2 38.99,6.35 40.32,7.68 52.7,7.68 53.02,8 J1.2 J2.2 64.77,8 S2.4 68.58,10.54 69.22,11.18 69.22,13.65 68.58,14.29 66.04,14.29 65.41,14.92 v65.41,15.62
SEL
  Bottom 0.406: IC1.3 IC1.2 140.3,24.77 141.25,23.81 144.11,23.81 144.75,23.18 JP1.2
TX
  Bottom 0.406: IC1.4 135.22,24.77 136.17,23.81 140.3,23.81 140.94,23.18 143.79,23.18 144.43,22.54 144.43,20.95 144.75,20.64 JP1.1
VCC  (via drill 0.6 pad 1.42)
  Top 0.406: v66.67,16.89 v66.67,24.51
  Top 0.61: v131.41,34.61 v131.41,25.72
  Bottom 0.406: R3.1 131.41,21.27 132.04,20.64 142.21,20.64 142.84,20 IC1.8 142.84,16.51 144.43,14.92 144.75,14.92 145.06,14.61 C1.1
  Bottom 0.61: 84.14,68.9 C8.1 IC2.8 | 84.14,68.9 80.93,68.9 80.93,47.62 JP6.1 71.12,40.96 71.12,40.95 70.48,40.31 70.48,27.68 67.31,24.51 v66.67,24.51 62.23,24.51 61.91,24.19 61.91,20.7 60.64,19.43 36.83,19.43 35.56,20.7 30.8,20.7 | 91.76,80.33 85.06,80.33 84.1,79.38 84.1,68.93 84.14,68.9 | 91.76,80.33 106.68,80.33 | 106.68,80.33 122.24,80.33 | 122.24,80.33 137.48,80.33 | 137.48,80.33 146.01,80.33 148.24,78.11 148.24,35.56 147.28,34.61 v131.41,34.61 | v131.41,25.72 R3.1 | R13.2 J2.3 J1.3 53.02,5.46 51.75,6.73 44.77,6.73 44.07,6.03 X16.3 | 30.8,20.7 26.04,20.7 26.04,20.71 26.04,14.99 26.99,14.04 IC4.3 | R13.2 67.31,8 70.48,11.18 70.48,13.97 69.22,15.24 67.31,15.24 66.67,15.88 v66.67,16.89 | R14.2 R13.2 | IC3.OUT 26.35,31.75 27.62,33.02 32.7,33.02 33.34,32.38 C10.1 C11.+ 33.33,20.71 30.8,20.7 | X1.2 91.68,80.25 91.76,80.33 | X2.2 106.91,80.1 106.68,80.33 | X3.2 122.16,80.25 122.24,80.33 | X4.2 137.4,80.25 137.48,80.33

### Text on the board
Bottom: IO-PWB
